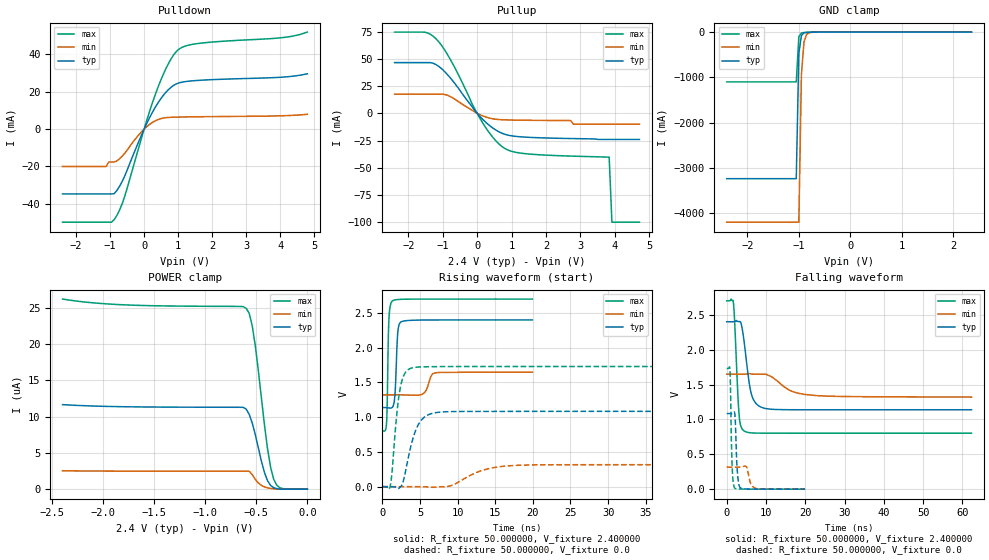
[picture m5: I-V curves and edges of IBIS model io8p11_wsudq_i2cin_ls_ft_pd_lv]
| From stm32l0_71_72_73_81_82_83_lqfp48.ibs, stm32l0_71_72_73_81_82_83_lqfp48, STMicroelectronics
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|   Model io8p11_wsudq_i2cin_ls_ft_pd_lv
[Model]  io8p11_wsudq_i2cin_ls_ft_pd_lv
Model_type I/O
Polarity   Non-Inverting
Enable   Active-Low
Vinl =   0.720000V
Vinh =   1.680000V
Vmeas =  1.200000V
Cref =   50.000000pF
Rref =   100.000000M
Vref =   0.0V
C_comp   2.943600pF   2.919700pF   2.965100pF
[Temperature Range]   25.000000   0.105000k   -40.000000
[Pullup Reference]   2.400000V   1.650000V   2.700000V
[Pulldown Reference]   0.0V   0.0V   0.0V
[POWER Clamp Reference]   2.400000V   1.650000V   2.700000V
[GND Clamp Reference]   0.0V   0.0V   0.0V
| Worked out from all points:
|   slope of the pulldown table from 0 to 0.36 V, typ, clamps not added: 28.5 ohm
|   slope of the pullup table from 0 to 0.36 V, typ, clamps not added: 32.2 ohm
|   GND clamp passes 1 mA (typ) near -0.64 V on its own axis
|   rising waveform, R_fixture 50.000000, V_fixture 2.400000: 20-80 % time 288ps typ, 643ps min, 198ps max; typ from 1.14 V to 2.4 V
|   rising waveform, R_fixture 50.000000, V_fixture 0.0: 20-80 % time 1.59ns typ, 3.84ns min, 930ps max; typ from 0 V to 1.08 V
|   falling waveform, R_fixture 50.000000, V_fixture 2.400000: 20-80 % time 1.81ns typ, 5.37ns min, 921ps max; typ from 2.4 V to 1.14 V
|   falling waveform, R_fixture 50.000000, V_fixture 0.0: 20-80 % time 489ps typ, 866ps min, 385ps max; typ from 1.08 V to 0 V
[Pulldown]
|Voltage   I(typ)   I(min)   I(max)
-2.4V     -34.7mA    -20mA      -49.82mA
-1.12V    -34.7mA    -20mA      -49.82mA
-1.04V    -34.7mA    -17.6mA    -49.82mA
-880mV    -34.55mA   -17.6mA    -48.46mA
-560mV    -24.65mA   -12.68mA   -35.33mA
0V        326fA      0A         140fA
400mV     13.84mA    5.066mA    22.03mA
720mV     21.25mA    6.254mA    35.26mA
1.04V     24.83mA    6.464mA    43.03mA
1.6V      26.11mA    6.627mA    45.88mA
4V        27.76mA    7.125mA    48.88mA
4.8V      29.63mA    7.94mA     51.96mA
[Pullup]
|Voltage   I(typ)   I(min)   I(max)
-2.4V     46.57mA    17.61mA    74.62mA
-1.52V    46.57mA    17.61mA    74.5mA
-1.2V     44.84mA    17.61mA    68.61mA
-720mV    30.25mA    14.38mA    46.12mA
-160mV    6.59mA     3.051mA    9.467mA
160mV     -5.477mA   -2.361mA   -8.695mA
480mV     -14.04mA   -5.167mA   -22.91mA
800mV     -19.2mA    -5.978mA   -32.18mA
1.52V     -22.07mA   -6.4mA     -37.42mA
3.84V     -24mA      -10mA      -40.2mA
3.92V     -24mA      -10mA      -100mA
4.72V     -24mA      -10mA      -100mA
[GND_clamp]
|Voltage   I(typ)   I(min)   I(max)
-2.4V     -3.237A    -4.198A    -1.1A
-1.05V    -3.237A    -4.198A    -1.1A
-1V       -475.8mA   -4.198A    -104.2mA
-950mV    -76.26mA   -935.5mA   -18.4mA
-900mV    -16.62mA   -212.9mA   -9.114mA
-850mV    -6.559mA   -50.96mA   -6.598mA
-800mV    -4.01mA    -13.82mA   -4.868mA
-650mV    -1.055mA   -1.198mA   -1.154mA
2.35V     52.69uA    50.02uA    36.84uA
[POWER_clamp]
|Voltage   I(typ)   I(min)   I(max)
-2.4V     11.64uA    2.525uA    26.17uA
-1.86V    11.37uA    2.488uA    25.42uA
-600mV    11.04uA    2.474uA    24.9uA
-570mV    10.3uA     2.473uA    24.21uA
-540mV    9.097uA    2uA        22.48uA
-510mV    7.497uA    1.35uA     19.73uA
-450mV    3.845uA    512.5nA    12.52uA
-390mV    1.154uA    175.5nA    5.528uA
-360mV    508.2nA    102.8nA    2.997uA
-330mV    204.4nA    60.39nA    1.375uA
-270mV    0A         0A         194.9nA
0V        0A         0A         0A
[Ramp]
| variable   typ   min   max
dV/dt_r  0.65004/1.58568n   0.18967/3.83970n   1.03746/0.92613n
dV/dt_f  0.75702/1.81197n   0.19614/5.35833n   1.13800/0.91870n
R_load = 50.000000
[Rising Waveform]
R_fixture= 50.000000
V_fixture= 2.400000
V_fixture_min= 1.650000
V_fixture_max= 2.700000
|time   V(typ)   V(min)   V(max)
0s        1.137V     1.32V      801.8mV
560.6ps   1.137V     1.32V      917.1mV
880.9ps   1.133V     1.32V      2.426V
1.321ns   1.141V     1.32V      2.671V
1.682ns   1.336V     1.32V      2.687V
2.082ns   2.252V     1.32V      2.693V
2.482ns   2.371V     1.32V      2.696V
5.365ns   2.398V     1.334V     2.699V
7.127ns   2.399V     1.639V     2.699V
19.94ns   2.399V     1.649V     2.699V
[Rising Waveform]
R_fixture= 50.000000
V_fixture= 0.0
V_fixture_min= 0.0
V_fixture_max= 0.0
|time   V(typ)   V(min)   V(max)
0s        -2.849uV   4.647uV    224.1uV
1.001ns   111.1uV    1.141uV    -13.27mV
1.251ns   -696.2uV   -1.732uV   168.1mV
2.002ns   -17.04mV   -4.864uV   1.132V
2.377ns   -8.141mV   10.77uV    1.419V
4.004ns   670.4mV    88.59uV    1.71V
5.506ns   993.5mV    -1.8mV     1.724V
8.383ns   1.078V     -262.1uV   1.728V
17.89ns   1.083V     307.2mV    1.729V
62.31ns   1.083V     316.1mV    1.729V
[Falling Waveform]
R_fixture= 50.000000
V_fixture= 2.400000
V_fixture_min= 1.650000
V_fixture_max= 2.700000
|time   V(typ)   V(min)   V(max)
0s        2.399V     1.649V     2.699V
1.752ns   2.398V     1.649V     2.655V
3.128ns   2.402V     1.649V     1.087V
3.754ns   2.355V     1.648V     881mV
4.63ns    2.026V     1.649V     828mV
5.756ns   1.512V     1.656V     810.1mV
6.381ns   1.345V     1.65V      806.6mV
9.51ns    1.161V     1.648V     802.4mV
19.89ns   1.138V     1.358V     801.8mV
62.31ns   1.137V     1.32V      801.8mV
[Falling Waveform]
R_fixture= 50.000000
V_fixture= 0.0
V_fixture_min= 0.0
V_fixture_max= 0.0
|time   V(typ)   V(min)   V(max)
0s        1.083V     316.1mV    1.729V
840.8ps   1.083V     316.1mV    1.709V
1.361ns   1.083V     316.1mV    370.1mV
2.002ns   1.1V       316.1mV    19.95mV
2.202ns   967.6mV    316.1mV    9.152mV
2.683ns   272.3mV    315.9mV    3.94mV
3.403ns   24.55mV    316mV      2.203mV
4.925ns   2.407mV    326.1mV    936.8uV
7.648ns   613.9uV    5.975mV    397.8uV
19.94ns   -2.849uV   4.647uV    224.1uV
